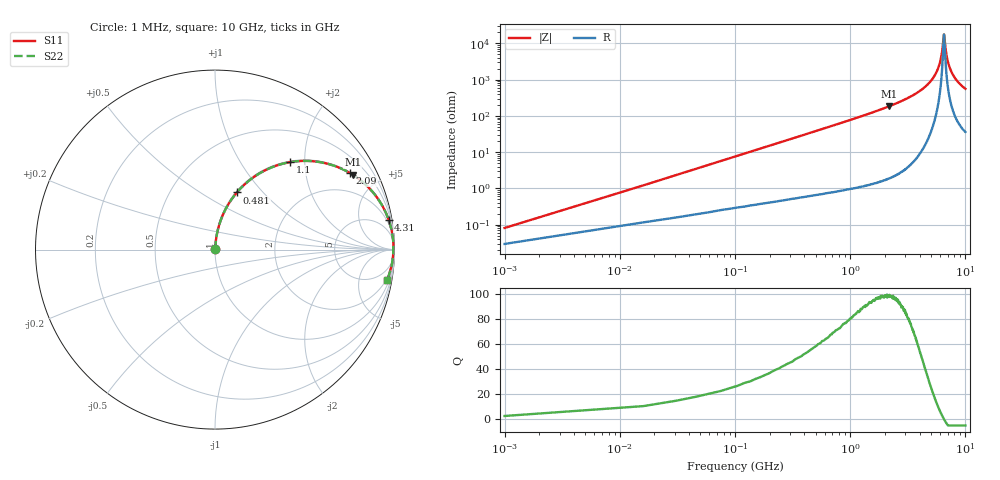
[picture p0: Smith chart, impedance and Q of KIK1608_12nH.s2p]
!version-2
!date-01.2022
!Series
# MHz S RI R 50
!Freq ReS11 ImS11 ReS21 ImS21 ReS12 ImS12 ReS22 ImS22
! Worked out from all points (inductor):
!   668 points, 1 MHz to 10 GHz, reference 50 ohm
!   read as one part in series: L = 12 nH near 46 MHz
!   highest Q = 98.4 at 2.16 GHz (marker M1), where L = 13.5 nH
!   self-resonance near 6.51 GHz
!   S11 on the Smith chart (normalised r, x): 1 MHz: 1.00, +0.00; 481 MHz: 1.01, +0.73; 1.1 GHz: 1.02, +1.70; 2.09 GHz: 1.04, +3.50; 4.31 GHz: 1, +12; 10 GHz: 2, -11
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1  0.000289 0.000754  0.9997 -0.000754  0.9997 -0.000754  0.000289 0.000754
61  0.00434 0.0457  0.9957 -0.0457  0.9957 -0.0457  0.00434 0.0457
106  0.00925 0.079  0.9907 -0.079  0.9907 -0.079  0.00925 0.079
241  0.0361 0.1746  0.9639 -0.1746  0.9639 -0.1746  0.0361 0.1746
481  0.1217 0.3183  0.8783 -0.3183  0.8783 -0.3183  0.1217 0.3183
1100  0.4206 0.4877  0.5794 -0.4877  0.5794 -0.4877  0.4206 0.4877
1670  0.6422 0.4742  0.3578 -0.4742  0.3578 -0.4742  0.6422 0.4742
2090  0.7521 0.4268  0.2479 -0.4268  0.2479 -0.4268  0.7521 0.4268
2160  0.7678 0.4172  0.2322 -0.4172  0.2322 -0.4172  0.7678 0.4172
3350  0.9184 0.2672  0.0816 -0.2672  0.0816 -0.2672  0.9184 0.2672
4310  0.9672 0.1674  0.0328 -0.1674  0.0328 -0.1674  0.9672 0.1674
5010  0.9843 0.1063  0.0157 -0.1063  0.0157 -0.1063  0.9843 0.1063
5570  0.9913 0.0639  0.00874 -0.0639  0.00874 -0.0639  0.9913 0.0639
5990  0.9938 0.0346  0.00623 -0.0346  0.00623 -0.0346  0.9938 0.0346
6260  0.9944 0.0168  0.0056 -0.0168  0.0056 -0.0168  0.9944 0.0168
6510  0.9944 0.00074  0.00562 -0.00074  0.00562 -0.00074  0.9944 0.00074
6560  0.9943 -0.00203  0.00567 0.00203  0.00567 0.00203  0.9943 -0.00203
6680  0.9941 -0.00931  0.0059 0.00931  0.0059 0.00931  0.9941 -0.00931
6900  0.9934 -0.0226  0.00662 0.0226  0.00662 0.0226  0.9934 -0.0226
7230  0.9917 -0.0413  0.00828 0.0413  0.00828 0.0413  0.9917 -0.0413
8340  0.9819 -0.0983  0.0181 0.0983  0.0181 0.0983  0.9819 -0.0983
10000  0.9586 -0.1695  0.0414 0.1695  0.0414 0.1695  0.9586 -0.1695
